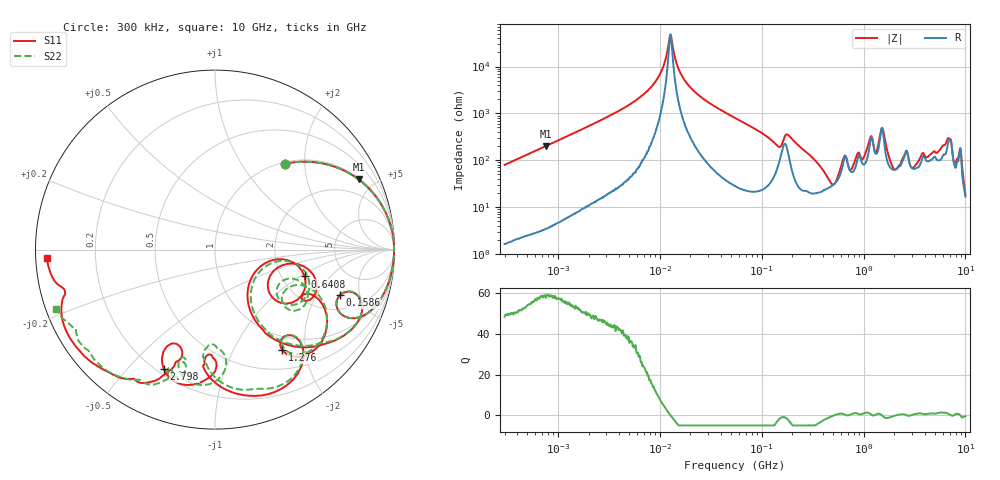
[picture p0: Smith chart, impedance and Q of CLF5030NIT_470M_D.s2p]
! S-Parameter Data Generated by TDK Corporation
! Copyright(C) 2019 TDK Corporation.
! All Rights Reserved.
! TDK P/N: CLF5030NIT-470M-D (Inductor)
! Property: L=47uH at 100kHz
! Size(LxWxT): 5.3x5x2.7mm
! Model Type: s2p (Touchstone File Format Version 1.0)
! Frequency: DC=Yes Start=0.3MHz Stop=10000MHz 802points Log-sweep
! Model Generated on May 10, 2019
! Port Assignments:
!  1 ---@@@--- 2
! Applicable Conditions:
!  Temperature = 25 degC
!  DC Bias Current = 0 A
!  Small Signal Operation
! Terms and conditions regarding TDK Simulation Models
! (1)This simulation model is being provided solely for informational purposes. Please refer to the specifications of the products in terms of detailed characteristics of such products.
! (2)In no event shall TDK Corporation of any of its subsidiaries be liable for any loss or damage arising, directly or indirectly,
!  From any information contained in this simulation model, including, but not limited to loss or damages arising from any inaccuracies, omissions or errors in connection with such information.
! (3)Any and all copyrights on this simulation model are owned by TDK Corporation.
!  Duplication or redistribution of this simulation model without prior written permission from TDK Corporation is prohibited.
! (4)This simulation model is subject to any modification or change without any prior notice.
! (5)Neither TDK Corporation nor any of its subsidiaries shall make any warranty, express or implied,
!  Including but not limited to the correctness, implied warranties of merchantability and fitness for a particular purpose with respect to this simulation models.
! (6)The use of this simulation model shall be deemed to have consented to the terms and conditions hereof.
# Hz S MA R 50
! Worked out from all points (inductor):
!   801 points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, 300 kHz to 10 GHz, reference 50 ohm
!   read as one part in series: L = 42 uH near 318.3 kHz
!   highest Q = 58.9 at 768.5 kHz (marker M1), where L = 42 uH
!   self-resonance near 12.73 MHz
!   S11 on the Smith chart (normalised r, x): 300 kHz: 1.03, +1.59; 158.6 MHz: 2.88, -3.24; 640.8 MHz: 2.67, -1.10; 1.276 GHz: 0.77, -1.59; 2.798 GHz: 0.23, -0.64; 10 GHz: 0.03, -0.03
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300000  0.6162 50.8  0.7751 -38.0  0.7752 -38.0  0.6161 50.9
768539  0.8907 26.0  0.4395 -63.0  0.4395 -63.0  0.8907 26.0
1713600  0.9726 12.3  0.214 -76.6  0.214 -76.6  0.9727 12.3
9671944  0.998 0.6  0.01688 -83.3  0.01688 -83.3  0.998 0.6
1.289893e7  0.9979 -0.6  0.002194 18.2  0.002197 18.9  0.9979 -0.6
1.49005e7  0.9977 -1.1  0.00961 75.8  0.009627 75.8  0.9978 -1.1
1.899897e7  0.9973 -2.2  0.02459 82.4  0.02459 82.4  0.9973 -2.2
5.477226e7  0.988 -9.3  0.1231 78.7  0.1231 78.7  0.9881 -9.3
1.585658e8  0.7412 -20.0  0.3284 25.1  0.3284 25.1  0.7401 -19.9
3.126428e8  0.735 -47.8  0.5743 33.7  0.5742 33.7  0.7341 -47.0
5.285151e8  0.2567 -37.4  0.7421 -16.1  0.7421 -16.1  0.275 -35.8
6.407886e8  0.5213 -16.7  0.4775 -36.3  0.4776 -36.3  0.5418 -16.6
8.299813e8  0.4736 -10.0  0.5413 -50.0  0.5415 -50.0  0.5151 -20.7
1.276148e9  0.6739 -56.2  0.32 -40.2  0.3201 -40.3  0.6725 -55.1
1.547353e9  0.8593 -64.6  0.1305 -36.5  0.1302 -36.4  0.8388 -65.5
1.767019e9  0.7825 -85.5  0.3317 -23.1  0.3317 -23.1  0.7633 -84.6
2.264206e9  0.6011 -91.3  0.4035 -72.9  0.4031 -72.9  0.5294 -93.3
2.798208e9  0.7253 -113.1  0.2731 -66.8  0.2724 -66.8  0.75 -101.2
4.399376e9  0.7817 -113.3  0.2139 -129.2  0.2139 -129.3  0.7566 -109.6
5.930102e9  0.8992 -129.3  0.0837 -171.2  0.08316 -171.2  0.8988 -130.1
8.770142e9  0.876 -166.0  0.01621 -146.3  0.01624 -147.9  0.9364 -156.4
1e10  0.9382 -177.0  0.0379 -84.5  0.03777 -84.4  0.9438 -159.5
